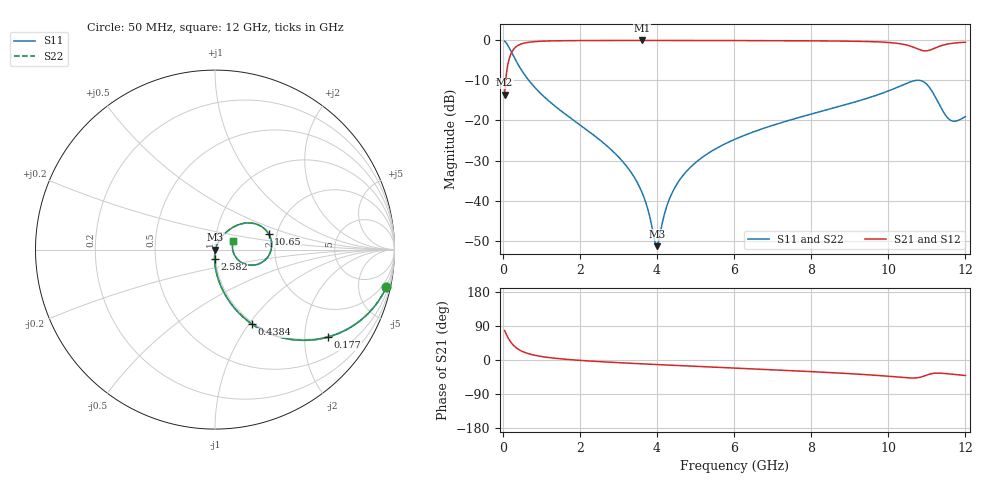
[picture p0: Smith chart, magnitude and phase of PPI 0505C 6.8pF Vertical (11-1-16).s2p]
# GHz S MA R 50
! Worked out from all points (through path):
!   1601 points, 50 MHz to 12 GHz, reference 50 ohm
!   highest |S21| = -0.02 dB at 3.613 GHz (marker M1); lowest = -13.6 dB at 50 MHz (marker M2)
!   group delay of S21, straight-line fit = 15.2 ps
!   lowest |S11| = -51.4 dB at 3.994 GHz (marker M3), VSWR 1.01, Z = 50.3 - j0.0587 ohm
!   |S11| at or under -10 dB: 678.9 MHz to 10.71 GHz (10.04 GHz wide, 176 % of centre); 10.82 GHz to end of sweep
!   |S22| runs from -51.4 to -0.2 dB; largest |S21 - S12| = 0
!   S11 on the Smith chart (normalised r, x): 50 MHz: 0.98, -9.20; 177 MHz: 0.98, -2.59; 438.4 MHz: 0.98, -1.04; 2.582 GHz: 0.99, -0.11; 10.65 GHz: 1.81, +0.35; 12 GHz: 1.22, +0.11
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0.05  0.9777 -12.3  0.21 77.7  0.21 77.7  0.9777 -12.3
0.1769688  0.7953 -37.8  0.6057 52.2  0.6057 52.2  0.7953 -37.8
0.2964688  0.6153 -52.9  0.7875 37.1  0.7875 37.1  0.6153 -52.9
0.438375  0.4645 -63.5  0.8846 26.4  0.8846 26.4  0.4645 -63.5
0.9089063  0.2366 -78.7  0.9702 10.9  0.9702 10.9  0.2366 -78.7
2.044156  0.08526 -90.0  0.9943 -1.3  0.9943 -1.3  0.08526 -90.0
2.581906  0.05399 -92.4  0.9962 -4.7  0.9962 -4.7  0.05399 -92.4
3.209281  0.02701 -93.0  0.997 -8.1  0.997 -8.1  0.02701 -93.0
3.612594  0.01269 -88.5  0.9971 -10.2  0.9971 -10.2  0.01269 -88.5
3.7545  0.008121 -82.1  0.9971 -10.9  0.9971 -10.9  0.008121 -82.1
3.9935  0.0027 -12.5  0.997 -12.0  0.997 -12.0  0.0027 -12.5
4.038312  0.003045 14.7  0.997 -12.2  0.997 -12.2  0.003045 14.7
4.29225  0.009546 59.5  0.9969 -13.4  0.9969 -13.4  0.009546 59.5
4.643281  0.01965 66.3  0.9966 -15.1  0.9966 -15.1  0.01965 66.3
5.203437  0.03542 67.2  0.9959 -17.6  0.9959 -17.6  0.03542 67.2
6.025  0.05835 65.1  0.9943 -21.4  0.9943 -21.4  0.05835 65.1
8.019156  0.1209 56.5  0.9865 -30.8  0.9865 -30.8  0.1209 56.5
10.01331  0.2347 39.3  0.9403 -43.0  0.9403 -43.0  0.2347 39.3
10.64816  0.3113 16.5  0.823 -47.6  0.823 -47.6  0.3113 16.5
11.00666  0.2802 -13.0  0.7407 -39.5  0.7407 -39.5  0.2802 -13.0
11.59669  0.102 -6.8  0.9097 -36.9  0.9097 -36.9  0.102 -6.8
12  0.1118 24.4  0.9473 -40.9  0.9473 -40.9  0.1118 24.4
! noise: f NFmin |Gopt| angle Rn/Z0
0.05  0.0005376  0.9054  1.549  0.001246
1.372  0.004806  0.7221  4.609  0.003423
2.701  0.007841  0.6744  8.366  0.004619
4.031  0.0106  0.6475  12.12  0.005644
5.36  0.01337  0.6333  15.83  0.006732
6.682  0.01655  0.6329  19.48  0.008246
8.012  0.02149  0.658  23.19  0.01153
9.341  0.0348  0.7431  27.14  0.02572
10.67  0.134  0.9168  31.3  0.3299
12  0.07483  0.8406  34.98  0.09055
